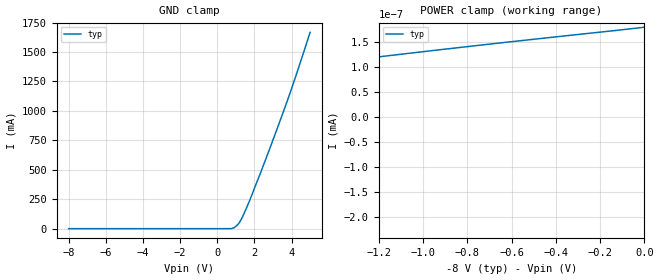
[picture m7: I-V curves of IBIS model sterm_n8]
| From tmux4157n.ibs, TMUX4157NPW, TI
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| sterm_n8
[Model]   sterm_n8
Model_type   Terminator
|   typ   min   max
C_comp   6.976543e-12   NA   NA
[Voltage Range]   -8   NA   NA
[Temperature Range]   27   NA   NA
[Power Clamp Reference]   -8   NA   NA
[GND Clamp Reference]   0   NA   NA
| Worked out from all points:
|   POWER clamp passes 1 mA (typ) near -8.76 V on its own axis
[GND Clamp]
|   Voltage   I(typ)   I(min)   I(max)
-8V       -502.5pA   NA         NA
535.4mV   13.79uA    NA         NA
798mV     1.378mA    NA         NA
929.3mV   9.875mA    NA         NA
1.192V    51.35mA    NA         NA
1.323V    88.13mA    NA         NA
1.717V    228.7mA    NA         NA
2.374V    491.7mA    NA         NA
3.03V     765.5mA    NA         NA
3.818V    1.106A     NA         NA
4.212V    1.287A     NA         NA
5V        1.667A     NA         NA
[POWER Clamp]
|   Voltage   I(typ)   I(min)   I(max)
-13V      -1.823A    NA         NA
-5.909V   -237.3pA   NA         NA
-5.778V   -223.4pA   NA         NA
-4.99V    -145.3pA   NA         NA
-4.465V   -98.47pA   NA         NA
-3.808V   -45.18pA   NA         NA
-3.152V   2.829pA    NA         NA
-2.495V   46.19pA    NA         NA
-1.707V   92.96pA    NA         NA
-919.2mV  135pA      NA         NA
0V        179.7pA    NA         NA
